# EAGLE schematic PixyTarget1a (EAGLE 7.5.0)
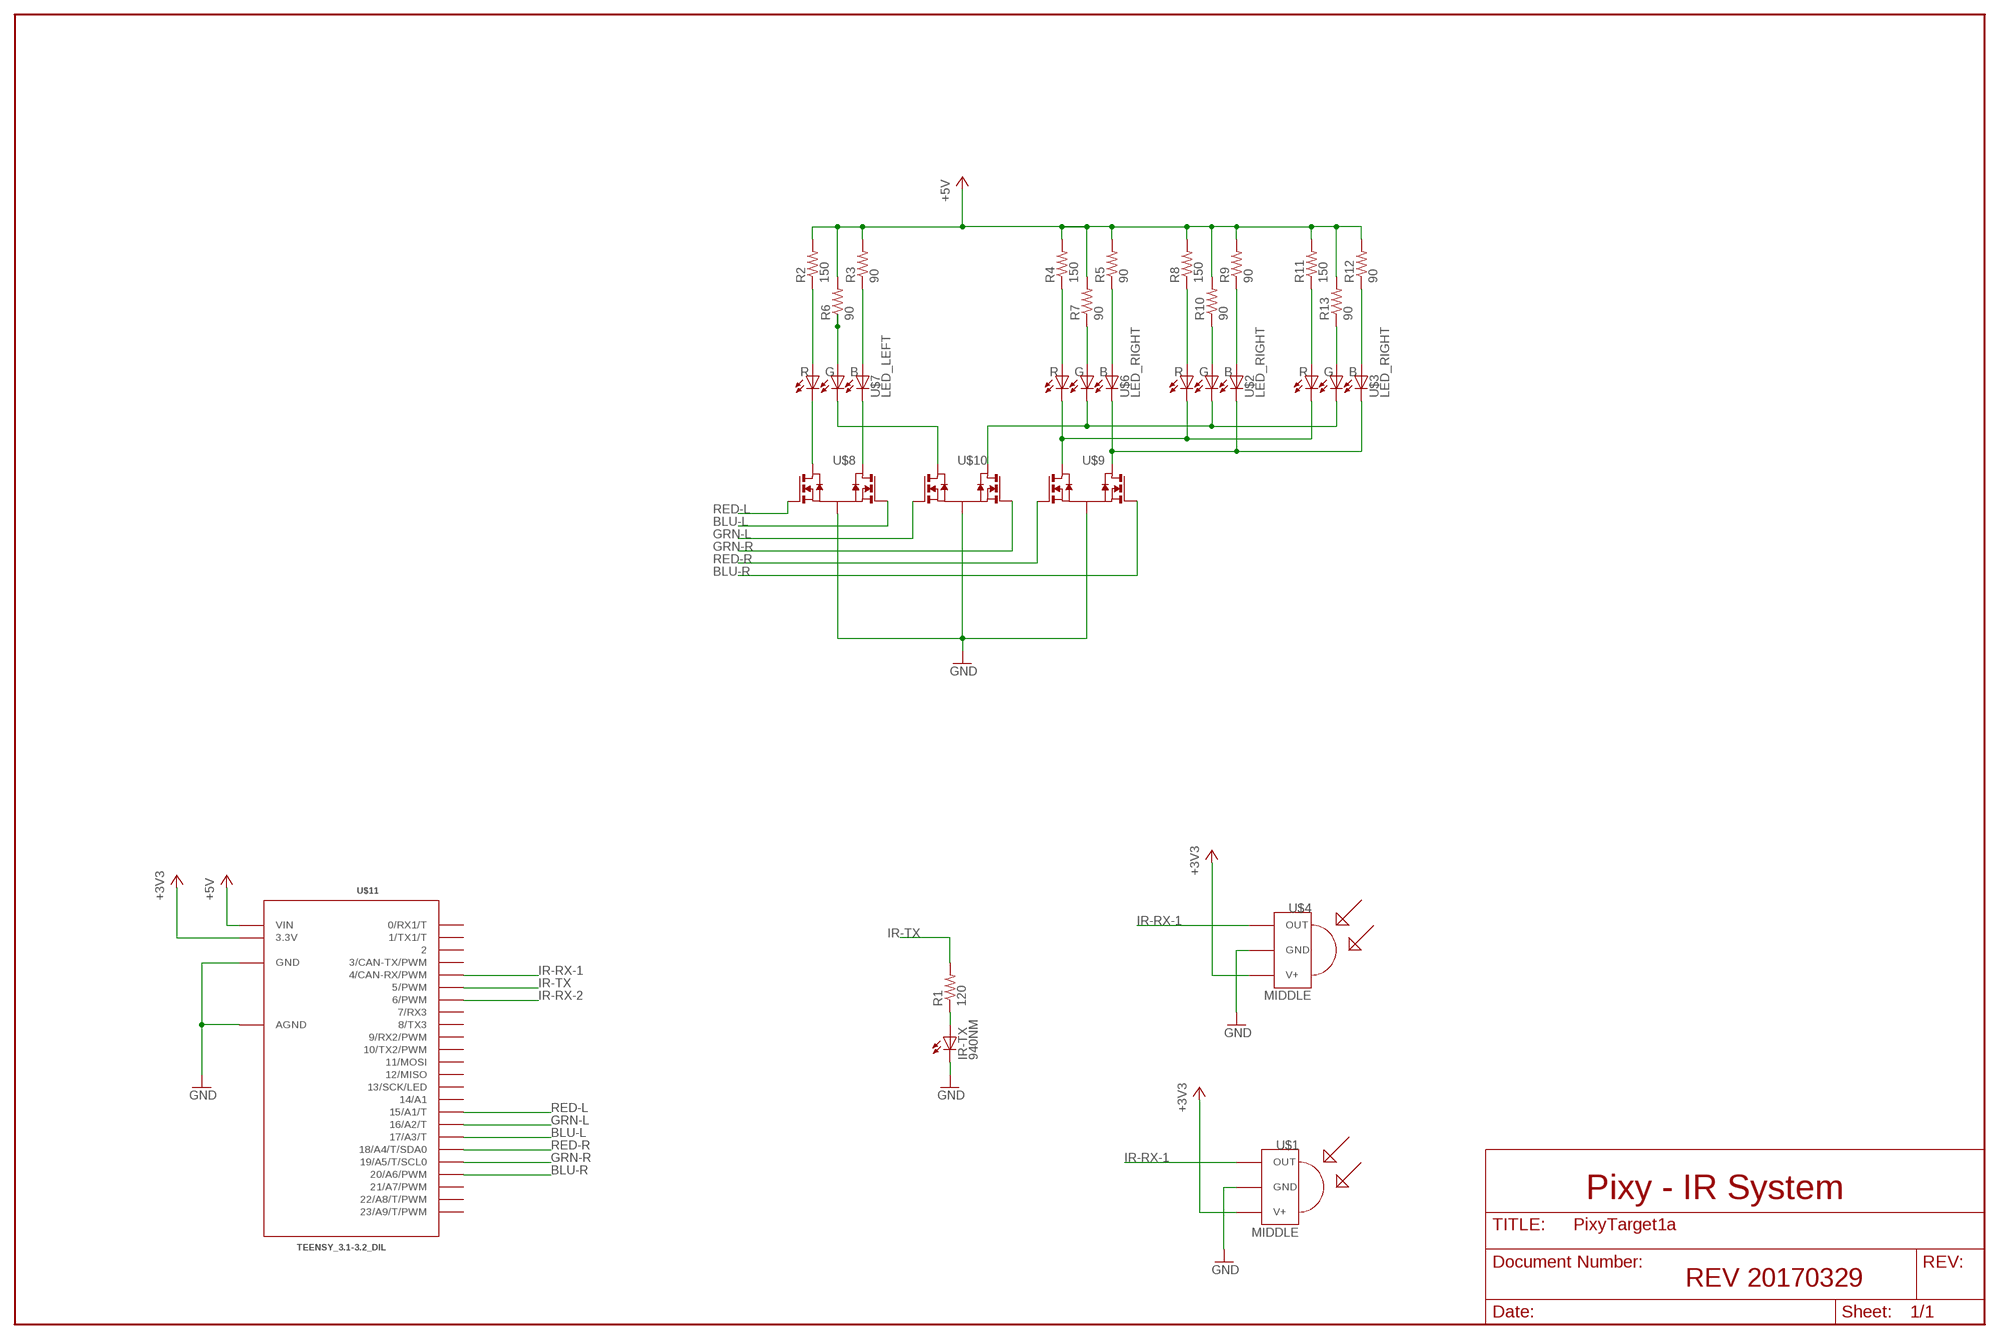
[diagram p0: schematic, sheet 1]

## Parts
IR-TX  940NM  LED5MM  [LED5MM]
R1  120  R-US_R1206  [R1206]
R2  150  R-US_R1206  [R1206]
R3  90  R-US_R1206  [R1206]
R4  150  R-US_R1206  [R1206]
R5  90  R-US_R1206  [R1206]
R6  90  R-US_R1206  [R1206]
R7  90  R-US_R1206  [R1206]
R8  150  R-US_R1206  [R1206]
R9  90  R-US_R1206  [R1206]
R10  90  R-US_R1206  [R1206]
R11  150  R-US_R1206  [R1206]
R12  90  R-US_R1206  [R1206]
R13  90  R-US_R1206  [R1206]
U$1  MIDDLE  TSOP3X  [TSOP18XX]
U$2  LED_RIGHT  LED_RGB_6SMD  [6-PLCC]
U$3  LED_RIGHT  LED_RGB_6SMD  [6-PLCC]
U$4  MIDDLE  TSOP3X  [TSOP18XX]
U$6  LED_RIGHT  LED_RGB_6SMD  [6-PLCC]
U$7  LED_LEFT  LED_RGB_6SMD  [6-PLCC]
U$8  QS5K2TR  [SOT-23-5]
U$9  QS5K2TR  [SOT-23-5]
U$10  QS5K2TR  [SOT-23-5]
U$11  TEENSY_3.1-3.2_DIL  [TEENSY_3.0-3.2&LC_DIL]

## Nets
+3V3: U$1.VCC(V+) U$4.VCC(V+) U$11.3.3V
+5V: R2.2 R3.2 R4.2 R5.2 R6.2 R7.2 R8.2 R9.2 R10.2 R11.2 R12.2 R13.2 U$11.VIN
BLU-L: U$8.3(G2) U$11.17/A3(17/A3/T)
BLU-R: U$9.3(G2) U$11.20/A6(20/A6/PWM)
GND [ground]: IR-TX.K(C) U$1.GND U$4.GND U$8.2(S) U$9.2(S) U$10.2(S) U$11.AGND U$11.GND
GRN-L: U$10.1(G1) U$11.16/A2(16/A2/T)
GRN-R: U$10.3(G2) U$11.19/A5(19/A5/T/SCL0)
IR-RX-1: U$1.OUT U$4.OUT U$11.4(4/CAN-RX/PWM)
IR-RX-2: U$11.6(6/PWM)
IR-TX: R1.2 U$11.5(5/PWM)
N$1: R8.1 U$2.P$1(A1)
N$2: R9.1 U$2.P$3(A3)
N$3: R2.1 U$7.P$1(A1)
N$4: R3.1 U$7.P$3(A3)
N$5: R6.1 U$7.P$2(A2)
N$6: U$7.P$5(C2) U$10.5(D1)
N$7: R10.1 U$2.P$2(A2)
N$8: U$2.P$6(C1) U$3.P$6(C1) U$6.P$6(C1) U$9.5(D1)
N$10: IR-TX.A R1.1
N$11: U$2.P$5(C2) U$3.P$5(C2) U$6.P$5(C2) U$10.4(D2)
N$12: R11.1 U$3.P$1(A1)
N$13: R12.1 U$3.P$3(A3)
N$14: R13.1 U$3.P$2(A2)
N$19: U$7.P$4(C3) U$8.4(D2)
N$20: U$7.P$6(C1) U$8.5(D1)
N$25: R4.1 U$6.P$1(A1)
N$26: R5.1 U$6.P$3(A3)
N$28: R7.1 U$6.P$2(A2)
N$30: U$2.P$4(C3) U$3.P$4(C3) U$6.P$4(C3) U$9.4(D2)
RED-L: U$8.1(G1) U$11.15/A1(15/A1/T)
RED-R: U$9.1(G1) U$11.18/A4(18/A4/T/SDA0)
Unconnected: U$11.0(0/RX1/T) U$11.1(1/TX1/T) U$11.2 U$11.3(3/CAN-TX/PWM) U$11.7(7/RX3) U$11.8(8/TX3) U$11.9(9/RX2/PWM) U$11.10(10/TX2/PWM) U$11.11(11/MOSI) U$11.12(12/MISO) U$11.13(13/SCK/LED) U$11.14/A0(14/A1) U$11.21/A7(21/A7/PWM) U$11.22/A8(22/A8/T/PWM) U$11.23/A9(23/A9/T/PWM)

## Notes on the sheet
- Pixy - IR System
- REV 20170329

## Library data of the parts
IR-TX = led:LED: LED
R1-R13 = resistor:R-US_: RESISTOR, American symbol
U$1 U$4 = _Loper:TSOP3X: IR Receiver and Demodulator
U$2 U$3 U$6 U$7 = _Loper:LED_RGB_6SMD
U$8-U$10 = _Loper:QS5K2TR: MOSFET 2N-CH
U$11 = Teensy_3_and_LC_Series_Boards_v1.4:TEENSY_3.1-3.2_DIL: Teensy 3.1 or 3.2 in a DIL Layout.

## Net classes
0 default: width 0.406 mm
1 ground: width 0.61 mm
